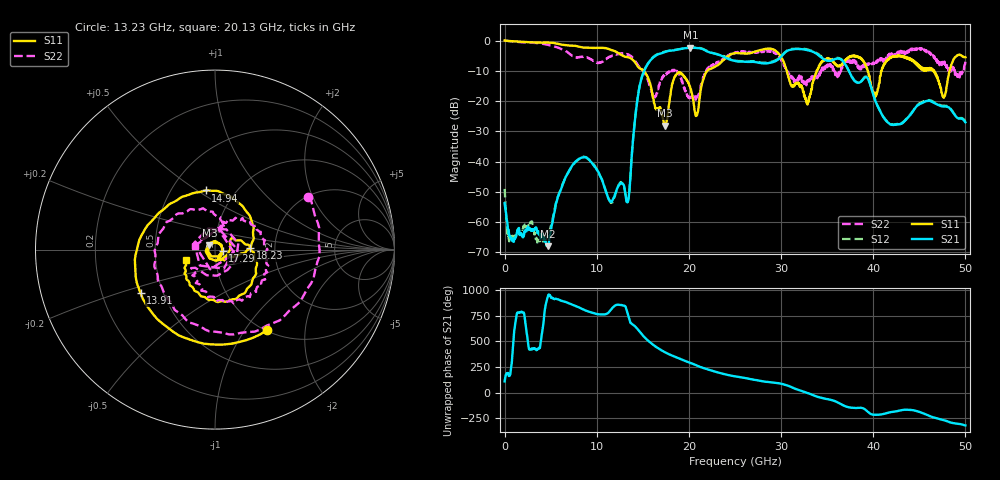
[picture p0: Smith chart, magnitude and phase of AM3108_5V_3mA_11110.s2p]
# Hz S DB R 50.0
!freq dBS11 angS11 dBS21 angS21 dBS12 angS12 dBS22 angS22
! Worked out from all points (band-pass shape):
!   1601 points, 10 MHz to 50 GHz, reference 50 ohm
!   highest |S21| = -2.31 dB at 20.16 GHz (marker M1); lowest = -68.0 dB at 4.697 GHz (marker M2)
!   |S21| within 3 dB of the highest: 16.25 GHz to 23.76 GHz (7.518 GHz wide, 37.6 % of centre); 30.01 GHz to 34.26 GHz (4.244 GHz wide, 13.2 % of centre)
!   lowest |S11| = -28.2 dB at 17.41 GHz (marker M3), VSWR 1.08, Z = 46.9 + j2.18 ohm
!   |S11| at or under -10 dB: 15.11 GHz to 21.99 GHz (6.875 GHz wide, 37.1 % of centre); 30.63 GHz to 33.86 GHz (3.232 GHz wide, 10 % of centre); 46.62 GHz to 48.29 GHz (1.668 GHz wide, 3.52 % of centre)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
!   |S22| runs from -19.5 to 0.1 dB; largest |S21 - S12| = 0.025
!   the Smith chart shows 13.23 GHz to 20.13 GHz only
!   S11 on the Smith chart (normalised r, x): 13.23 GHz: 1.01, -1.28; 13.91 GHz: 0.37, -0.24; 14.94 GHz: 0.73, +0.54; 17.29 GHz: 1.09, -0.01; 18.23 GHz: 1.49, +0.02; 20.13 GHz: 0.72, -0.09
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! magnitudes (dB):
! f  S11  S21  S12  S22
! 10 MHz  0.1  -53.7  -49.0  0.1
! 541.1 MHz  -0.1  -64.7  -65.4  -0.2
! 4.697 GHz  -0.6  -68.0  -64.0  -1.4
! 8.352 GHz  -2.2  -38.7  -38.5  -5.3
! 13.23 GHz  -5.4  -53.1  -52.9  -4.5
! 13.91 GHz  -6.4  -33.8  -33.7  -5.8
! 14.94 GHz  -9.5  -11.7  -11.5  -9.6
! 16.69 GHz  -22.7  -4.5  -4.3  -15.9
! 17.29 GHz  -27.4  -3.9  -3.7  -11.8
! 17.41 GHz  -28.2  -3.8  -3.6  -11.5
! 18.23 GHz  -14.2  -3.2  -3.1  -9.9
! 20.13 GHz  -15.3  -2.3  -2.2  -18.8
! 20.16 GHz  -15.8  -2.3  -2.2  -19.0
! 20.85 GHz  -24.7  -2.4  -2.3  -18.5
! 21.91 GHz  -10.3  -3.5  -3.3  -9.6
! 25 GHz  -4.1  -6.7  -6.6  -4.1
! 33.35 GHz  -15.8  -3.5  -3.4  -12.7
! 38 GHz  -5.0  -13.4  -13.3  -6.6
! 40.22 GHz  -18.6  -19.8  -19.7  -7.6
! 41.69 GHz  -6.0  -27.3  -27.2  -5.3
! 47.66 GHz  -18.9  -21.8  -21.5  -7.6
! 50 GHz  -5.5  -27.0  -26.6  -6.8
